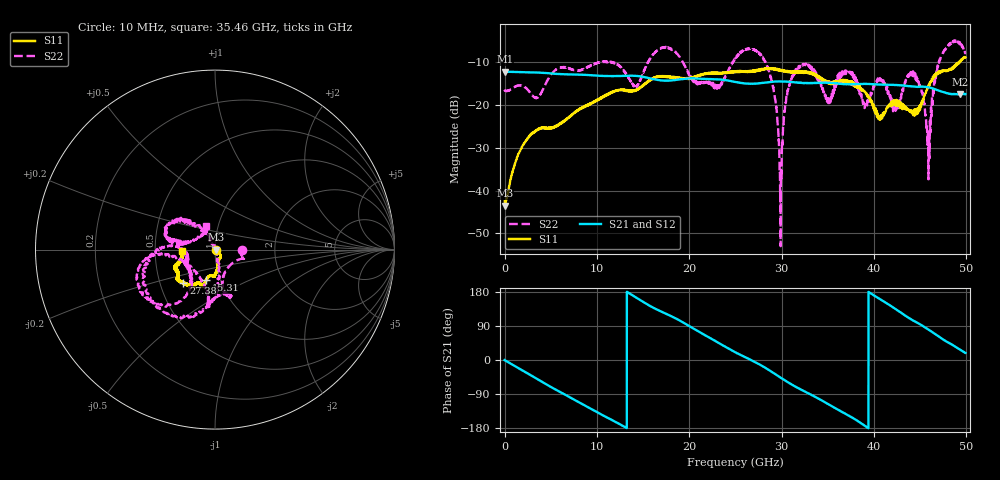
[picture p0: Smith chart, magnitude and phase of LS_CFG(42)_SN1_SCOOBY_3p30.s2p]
!Keysight Technologies,N5245B,MY58422026,A.13.80.08
!Date: Thursday, March 19, 2020 23:40:01
!Correction: S11(Full 2 Port(1,2))
!S21(Full 2 Port(1,2))
!S12(Full 2 Port(1,2))
!S22(Full 2 Port(1,2))
!S2P File: Measurements: S11, S21, S12, S22:
# Hz S DB R 50.0
!freq dBS11 angS11 dBS21 angS21 dBS12 angS12 dBS22 angS22
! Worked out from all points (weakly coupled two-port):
!   4991 points, 10 MHz to 49.91 GHz, reference 50 ohm
!   highest |S21| = -12.19 dB at 20 MHz (marker M1); lowest = -17.5 dB at 49.34 GHz (marker M2)
!   lowest |S11| = -43.5 dB at 30 MHz (marker M3), VSWR 1.01, Z = 50.7 - j0.0256 ohm
!   |S11| at or under -10 dB: start of sweep to 49.14 GHz; 49.15357 GHz to 49.23183 GHz (78.25 MHz wide, 0.159 % of centre); 49.30939 GHz to 49.32093 GHz (11.54 MHz wide, 0.0234 % of centre)
!   |S22| runs from -53.0 to -4.9 dB; largest |S21 - S12| = 0.0022
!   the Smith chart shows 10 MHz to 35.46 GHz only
!   S11 on the Smith chart (normalised r, x): 10 MHz: 1.01, -0.01; 15.31 GHz: 0.86, -0.30; 27.38 GHz: 0.66, -0.26; 35.46 GHz: 0.69, -0.01
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1e7  -42.54 -22.8  -12.19 -0.3  -12.18 -0.3  -16.42 0.0
2e7  -43.45 -7.2  -12.19 -0.4  -12.18 -0.4  -16.59 -0.5
3e7  -43.51 -2.2  -12.19 -0.5  -12.18 -0.5  -16.61 -1.0
2.71e9  -27.12 -46.3  -12.35 -38.3  -12.34 -38.3  -16.94 -23.2
8.33e9  -20.83 -80.2  -12.89 -115.5  -12.88 -115.4  -11.77 -85.3
1.531e10  -15.01 -106.4  -13.54 148.9  -13.53 149.0  -11.07 -174.9
1.665e10  -13.39 -107.7  -14.14 131.5  -14.13 131.5  -7.05 -164.5
2.299e10  -12.62 -119.9  -13.97 47.9  -13.97 48.0  -16.12 -163.3
2.496e10  -12.26 -124.8  -14.55 20.7  -14.54 20.8  -9.29 -175.0
2.738e10  -11.88 -133.8  -14.97 -8.7  -14.96 -8.6  -7.40 -116.6
2.906e10  -11.58 -142.8  -14.53 -33.1  -14.52 -33.0  -15.68 -84.9
2.989e10  -11.97 -144.6  -14.50 -46.5  -14.50 -46.3  -41.62 -5.1
3.093e10  -12.22 -147.0  -14.58 -62.2  -14.58 -62.0  -14.53 132.4
3.328e10  -12.57 -159.2  -14.84 -92.8  -14.84 -92.5  -11.43 168.1
3.546e10  -14.64 -177.1  -14.85 -122.1  -14.80 -121.7  -16.95 113.9
3.699e10  -14.55 172.5  -15.09 -143.1  -15.01 -143.2  -12.46 119.4
4.16e10  -20.00 102.0  -15.27 146.5  -15.30 146.3  -17.52 16.0
4.436e10  -21.08 57.2  -15.70 102.7  -15.72 102.7  -12.58 -23.9
4.591e10  -15.51 3.8  -15.84 80.4  -15.86 80.4  -37.36 -71.0
4.711e10  -12.10 7.4  -16.68 60.6  -16.70 60.8  -9.43 -101.8
4.934e10  -9.87 -18.7  -17.48 27.2  -17.50 27.4  -5.37 -35.4
4.991e10  -8.82 -16.2  -17.42 18.7  -17.44 18.7  -7.80 -21.1
